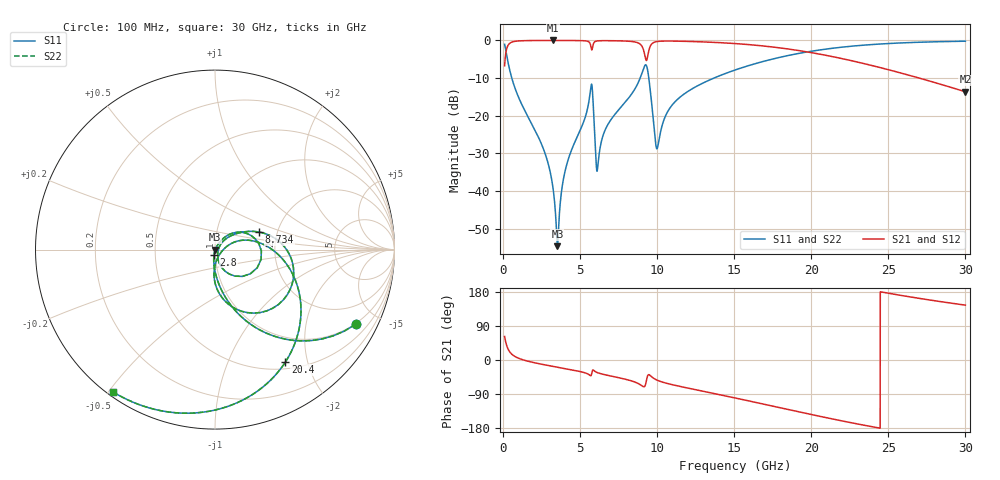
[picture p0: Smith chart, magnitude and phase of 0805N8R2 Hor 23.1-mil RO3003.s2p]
# GHz S MA R 50
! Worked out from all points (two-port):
!   3201 points, 100 MHz to 30 GHz, reference 50 ohm
!   highest |S21| = -0.02 dB at 3.23 GHz (marker M1); lowest = -13.6 dB at 30 GHz (marker M2)
!   |S21| within 3 dB of the highest: 192.1 MHz to 9.146 GHz (8.954 GHz wide, 192 % of centre); 9.441 GHz to 19.67 GHz (10.23 GHz wide, 70.3 % of centre)
!   lowest |S11| = -54.7 dB at 3.529 GHz (marker M3), VSWR 1.00, Z = 50.2 - j0.0629 ohm
!   |S11| at or under -10 dB: 565.3 MHz to 8.896 GHz (8.331 GHz wide, 176 % of centre); 9.457 GHz to 13.69 GHz (4.231 GHz wide, 36.6 % of centre)
!   |S22| runs from -54.7 to -0.2 dB; largest |S21 - S12| = 0
!   S11 on the Smith chart (normalised r, x): 100 MHz: 0.97, -3.78; 2.8 GHz: 0.99, -0.06; 8.734 GHz: 1.61, +0.34; 20.4 GHz: 0.60, -1.64; 30 GHz: 0.02, -0.51
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0.1  0.8873 -28.0  0.4607 62.0  0.4607 62.0  0.8873 -28.0
0.3709688  0.4574 -64.7  0.8887 25.2  0.8887 25.2  0.4574 -64.7
0.660625  0.2722 -77.6  0.9615 12.2  0.9615 12.2  0.2722 -77.6
2.800344  0.02832 -100.3  0.9979 -13.5  0.9979 -13.5  0.02832 -100.3
3.230156  0.01131 -98.0  0.9981 -16.8  0.9981 -16.8  0.01131 -98.0
3.529156  0.001849 -19.8  0.998 -19.0  0.998 -19.0  0.001849 -19.8
4.06175  0.01982 60.8  0.9975 -23.0  0.9975 -23.0  0.01982 60.8
5.089563  0.07037 54.8  0.9926 -31.3  0.9926 -31.3  0.07037 54.8
5.715594  0.2535 3.0  0.8011 -40.7  0.8011 -40.7  0.2535 3.0
6.15475  0.02194 17.9  0.986 -33.9  0.986 -33.9  0.02194 17.9
6.743406  0.07263 45.5  0.9916 -40.1  0.9916 -40.1  0.07263 45.5
8.733625  0.2651 21.6  0.9318 -61.3  0.9318 -61.3  0.2651 21.6
9.322281  0.4529 -47.7  0.547 -50.1  0.547 -50.1  0.4529 -47.7
9.565219  0.2053 -88.3  0.8477 -41.6  0.8477 -41.6  0.2053 -88.3
9.882906  0.04608 -69.1  0.9557 -51.0  0.9557 -51.0  0.04608 -69.1
10.06978  0.04184 -7.7  0.9705 -54.5  0.9705 -54.5  0.04184 -7.7
11.29381  0.163 18.7  0.977 -68.0  0.977 -68.0  0.163 18.7
15.05  0.404 -11.1  0.9076 -100.1  0.9076 -100.1  0.404 -11.1
20.03956  0.7197 -54.8  0.6859 -144.2  0.6859 -144.2  0.7197 -54.8
20.40397  0.739 -57.9  0.6652 -147.4  0.6652 -147.4  0.739 -57.9
25.01978  0.9089 -94.4  0.4073 176.1  0.4073 176.1  0.9089 -94.4
30  0.9755 -125.7  0.2078 144.8  0.2078 144.8  0.9755 -125.7
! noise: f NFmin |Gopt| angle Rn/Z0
0.1  0.0007095  0.9134  0.999  0.001805
3.417  0.005965  0.6892  18.46  0.00364
6.743  0.01454  0.7448  35.75  0.01039
10.06  0.04032  0.8576  52.64  0.0487
13.39  0.02246  0.6985  67.44  0.01022
16.7  0.02671  0.6951  81.37  0.01007
20.03  0.0338  0.7189  94.68  0.01127
23.35  0.04412  0.7561  107.6  0.01322
26.67  0.05976  0.8018  120.5  0.01599
30  0.08503  0.8509  133.5  0.01963
